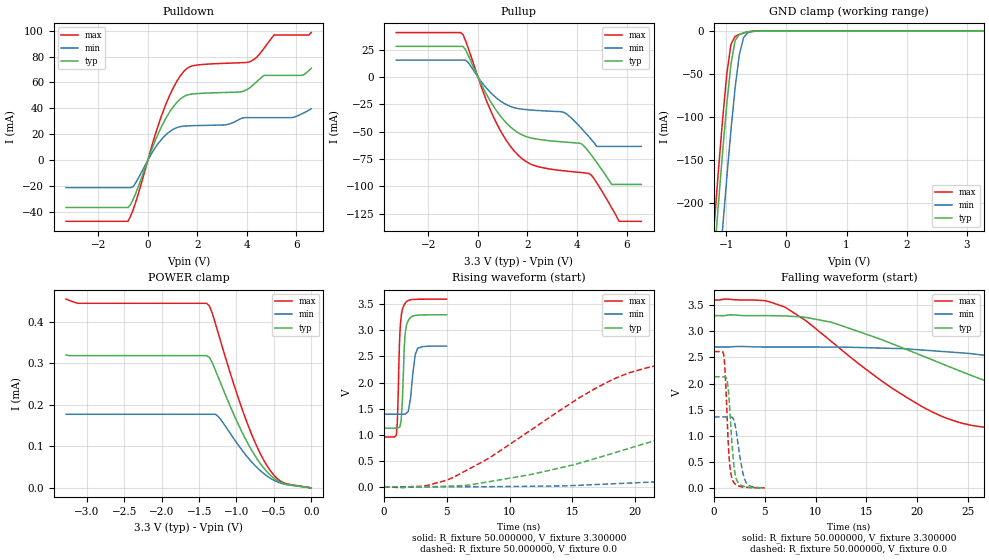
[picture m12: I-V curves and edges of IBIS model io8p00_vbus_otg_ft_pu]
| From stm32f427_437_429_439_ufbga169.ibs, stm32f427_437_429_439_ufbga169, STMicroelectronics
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|   Model io8p00_vbus_otg_ft_pu
[Model]  io8p00_vbus_otg_ft_pu
Model_type I/O
Polarity   Non-Inverting
Enable   Active-Low
Vinl =   0.990000V
Vinh =   2.310000V
Vmeas =  1.650000V
Cref =   50.000000pF
Rref =   100.000000M
Vref =   0.0V
C_comp   3.304800pF   3.199300pF   3.429300pF
[Temperature Range]   25.000000   0.125000k   -40.000000
[Pullup Reference]   3.300000V   2.700000V   3.600000V
[Pulldown Reference]   0.0V   0.0V   0.0V
[POWER Clamp Reference]   3.300000V   2.700000V   3.600000V
[GND Clamp Reference]   0.0V   0.0V   0.0V
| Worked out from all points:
|   slope of the pulldown table from 0 to 0.495 V, typ, clamps not added: 20.9 ohm
|   slope of the pullup table from 0 to 0.495 V, typ, clamps not added: 22.6 ohm
|   GND clamp passes 1 mA (typ) near -0.61 V on its own axis
|   rising waveform, R_fixture 50.000000, V_fixture 3.300000: 20-80 % time 222ps typ, 350ps min, 205ps max; typ from 1.12 V to 3.3 V
|   rising waveform, R_fixture 50.000000, V_fixture 0.0: 20-80 % time 19.2ns typ, 47.8ns min, 10.3ns max; typ from 0.001 V to 2.13 V
|   falling waveform, R_fixture 50.000000, V_fixture 3.300000: 20-80 % time 18.4ns typ, 37.8ns min, 11.3ns max; typ from 3.3 V to 1.12 V
|   falling waveform, R_fixture 50.000000, V_fixture 0.0: 20-80 % time 480ps typ, 675ps min, 386ps max; typ from 2.13 V to 0.001 V
[Pulldown]
|Voltage   I(typ)   I(min)   I(max)
-3.3V     -36.41mA   -21.08mA   -47.04mA
-800mV    -36.41mA   -21.08mA   -47.04mA
-600mV    -30.48mA   -20.53mA   -38.65mA
700mV     31.4mA     19.11mA    41.71mA
1.2V      45.15mA    25.37mA    61.75mA
1.6V      50.35mA    26.5mA     71.06mA
3.1V      52.28mA    27.26mA    74.76mA
4.1V      55.64mA    32.87mA    75.8mA
4.7V      65.47mA    32.87mA    86.49mA
5.1V      65.47mA    32.87mA    96.56mA
6.2V      65.47mA    35.57mA    96.56mA
6.6V      70.92mA    39.71mA    98.46mA
[Pullup]
|Voltage   I(typ)   I(min)   I(max)
-3.3V     28.01mA    15.42mA    40.63mA
-700mV    28.01mA    15.42mA    40.63mA
-400mV    20.31mA    13.47mA    26.93mA
600mV     -25.77mA   -16.23mA   -35.13mA
1.6V      -50.64mA   -28.8mA    -70.96mA
3.5V      -59.52mA   -32.65mA   -85.91mA
4.2V      -61.44mA   -47.48mA   -87.46mA
4.5V      -69.06mA   -55.12mA   -88.39mA
4.8V      -78.22mA   -63.5mA    -96.84mA
5.4V      -98.3mA    -63.5mA    -119.6mA
5.7V      -98.3mA    -63.5mA    -132mA
6.6V      -98.3mA    -63.5mA    -132mA
[GND_clamp]
|Voltage   I(typ)   I(min)   I(max)
-3.3V     -2.322A    -2.4A      -2.296A
-1.2V     -265.6mA   -356.2mA   -227.3mA
-1.13V    -202.8mA   -293mA     -164.3mA
-1.06V    -142.3mA   -231.2mA   -104.3mA
-990mV    -86.15mA   -171.7mA   -51mA
-920mV    -39.05mA   -115.6mA   -15.71mA
-850mV    -11.4mA    -65.74mA   -6.366mA
-780mV    -4.046mA   -27.6mA    -4.153mA
-710mV    -2.285mA   -7.882mA   -2.591mA
-640mV    -1.291mA   -2.274mA   -1.367mA
-570mV    -618uA     -909.9uA   -567.3uA
3.28V     0A         0A         0A
[POWER_clamp]
|Voltage   I(typ)   I(min)   I(max)
-3.28V    319.9uA    177.1uA    454.3uA
-3.12V    318.3uA    177.1uA    444.3uA
-1.4V     318.3uA    177.1uA    444.3uA
-1.36V    313.4uA    177.1uA    437.2uA
-1.28V    282.3uA    177.1uA    394.1uA
-1.24V    264.6uA    170.9uA    369.7uA
-920mV    131.9uA    89.38uA    187.2uA
-760mV    79.47uA    55.16uA    112.7uA
-640mV    48.78uA    35.06uA    68.06uA
-520mV    26.21uA    20.13uA    35uA
-400mV    12.52uA    10.84uA    14.88uA
0V        0A         0A         0A
[Ramp]
| variable   typ   min   max
dV/dt_r  1.27723/19.20156n   0.81633/47.97972n   1.56688/10.32038n
dV/dt_f  1.30500/18.34236n   0.78402/37.83839n   1.58713/11.31358n
R_load = 50.000000
[Rising Waveform]
R_fixture= 50.000000
V_fixture= 3.300000
V_fixture_min= 2.700000
V_fixture_max= 3.600000
|time   V(typ)   V(min)   V(max)
0s        1.125V     1.393V     954.7mV
991ps     1.127V     1.393V     1.005V
1.061ns   1.129V     1.393V     1.216V
1.281ns   1.172V     1.393V     2.997V
1.461ns   1.624V     1.392V     3.395V
1.552ns   2.219V     1.394V     3.46V
1.722ns   2.998V     1.398V     3.533V
2.032ns   3.224V     1.581V     3.582V
2.683ns   3.293V     2.658V     3.598V
4.985ns   3.3V       2.7V       3.6V
[Rising Waveform]
R_fixture= 50.000000
V_fixture= 0.0
V_fixture_min= 0.0
V_fixture_max= 0.0
|time   V(typ)   V(min)   V(max)
0s        1.088mV    1.043mV    1.136mV
5.506ns   17.46mV    2.756mV    178.8mV
12.01ns   253.1mV    12.25mV    1.141V
19.52ns   738.6mV    72.7mV     2.187V
25.03ns   1.126V     131.8mV    2.442V
32.53ns   1.609V     235.1mV    2.547V
46.05ns   1.987V     495.8mV    2.6V
76.58ns   2.113V     1.035V     2.612V
97.6ns    2.122V     1.214V     2.613V
249.2ns   2.13V      1.36V      2.613V
[Falling Waveform]
R_fixture= 50.000000
V_fixture= 3.300000
V_fixture_min= 2.700000
V_fixture_max= 3.600000
|time   V(typ)   V(min)   V(max)
0s        3.3V       2.7V       3.6V
6.507ns   3.298V     2.7V       3.497V
11.51ns   3.176V     2.697V     2.814V
22.02ns   2.414V     2.621V     1.409V
31.53ns   1.723V     2.432V     1.076V
37.04ns   1.462V     2.306V     1.035V
47.55ns   1.267V     2.056V     996.6mV
64.06ns   1.183V     1.71V      970.1mV
89.59ns   1.144V     1.514V     957.6mV
249.2ns   1.125V     1.393V     954.7mV
[Falling Waveform]
R_fixture= 50.000000
V_fixture= 0.0
V_fixture_min= 0.0
V_fixture_max= 0.0
|time   V(typ)   V(min)   V(max)
0s        2.13V      1.36V      2.613V
981ps     2.131V     1.36V      2.511V
1.151ns   2.121V     1.359V     1.98V
1.311ns   2.033V     1.359V     1.242V
1.491ns   1.669V     1.361V     562.1mV
1.812ns   732.9mV    1.346V     157.6mV
2.182ns   177.9mV    1.088V     59.17mV
2.573ns   61.71mV    563.1mV    28.51mV
3.033ns   25.97mV    155.9mV    14.27mV
4.985ns   1.088mV    1.043mV    1.136mV
